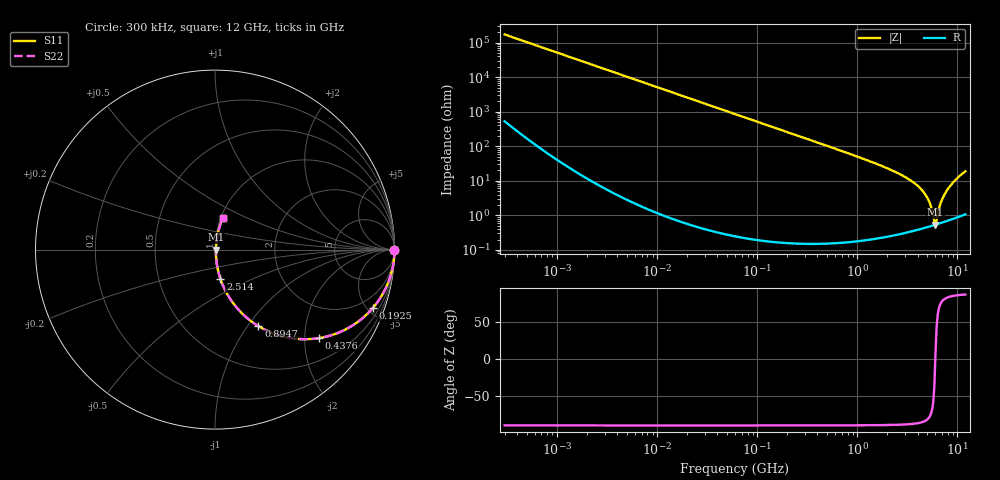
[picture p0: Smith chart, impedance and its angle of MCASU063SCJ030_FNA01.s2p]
! MCASU063SCJ030_FNA01  S-PARAMETER MODEL  ( Standard Model )
! Model Generated by TAIYO YUDEN Corporation (http://www.ty-top.com)
! Version 1.0
! TAIYO YUDEN Control No. 230609
! Copyright(c) 2023 TAIYO YUDEN CO.,LTD. All Rights Reserved.
! Product Description (link to TY-COMPAS)
! https://ds.yuden.co.jp/TYCOMPAS/or/detail?pn=MCASU063SCJ030BFNA01&u=M
! Products Name : Multilayer Ceramic Capacitors
! Characteristics :
!  Capacitance : 3 [pF] , Rated Voltage : 50 [V] , TCC : CJ / C0J
!  Case Size : 0.6 x 0.3 / 0.024 x 0.012 [mm/inch] , Thickness : 0.3 / 0.012 [mm/inch]
!  (Conditions: Temperature = 25 [degC] , DC Bias Voltage = 0 [V])
! External Node Assignments :
!  1  o---| |---o  2
! GND o---------o GND
! Frequency Range : 0.3MHz  -  12000MHz  [ 401 STEP ]
# MHZ S RI R 50
! Freq[MHz].  S11 Real  S11 Imag  S21 Real  S21 Imag  S12 Real  S12 Imag  S22 Real  S22 Imag
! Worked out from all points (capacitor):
!   401 points, 300 kHz to 12 GHz, reference 50 ohm
!   read as one part in series: C = 3.08 pF near 316.3 kHz
!   lowest |Z| = 538 mohm at 6.026 GHz (marker M1)
!   series resonance near 6.009 GHz, so ESL is about 230 pH
!   S11 on the Smith chart (normalised r, x): 300 kHz: open; 192.5 MHz: 1.00, -5.36; 437.6 MHz: 1.00, -2.35; 894.7 MHz: 1.00, -1.13; 2.514 GHz: 1.01, -0.34; 12 GHz: 1.02, +0.38
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0.3  1 -0.000581  2.12e-06 0.000581  2.12e-06 0.000581  1 -0.000581
1.769972  1 -0.00343  1.34e-05 0.00343  1.34e-05 0.00343  1 -0.00343
10.44266  0.9996 -0.0202  0.000413 0.0202  0.000413 0.0202  0.9996 -0.0202
60  0.9866 -0.1147  0.0134 0.1147  0.0134 0.1147  0.9866 -0.1147
192.4766  0.8776 -0.3274  0.1224 0.3274  0.1224 0.3274  0.8776 -0.3274
353.9943  0.6786 -0.4665  0.3214 0.4665  0.3214 0.4665  0.6786 -0.4665
437.5599  0.5794 -0.493  0.4206 0.493  0.4206 0.493  0.5794 -0.493
894.6982  0.2422 -0.4269  0.7578 0.4269  0.7578 0.4269  0.2422 -0.4269
2088.533  0.0473 -0.2066  0.9527 0.2066  0.9527 0.2066  0.0473 -0.2066
2514.07  0.0305 -0.1639  0.9695 0.1639  0.9695 0.1639  0.0305 -0.1639
3547.679  0.0123 -0.0934  0.9877 0.0934  0.9877 0.0934  0.0123 -0.0934
4502.883  0.00666 -0.0499  0.9933 0.0499  0.9933 0.0499  0.00666 -0.0499
5140.631  0.00536 -0.0268  0.9946 0.0268  0.9946 0.0268  0.00536 -0.0268
5420.343  0.00517 -0.0177  0.9948 0.0177  0.9948 0.0177  0.00517 -0.0177
5715.274  0.00516 -0.00868  0.9948 0.00868  0.9948 0.00868  0.00516 -0.00868
6026.253  0.00533 0.000513  0.9947 -0.000513  0.9947 -0.000513  0.00533 0.000513
6354.153  0.00568 0.00954  0.9943 -0.00954  0.9943 -0.00954  0.00568 0.00954
6699.894  0.00623 0.0191  0.9938 -0.0191  0.9938 -0.0191  0.00623 0.0191
7064.448  0.00702 0.0292  0.993 -0.0292  0.993 -0.0292  0.00702 0.0292
7854.144  0.0095 0.0515  0.9905 -0.0515  0.9905 -0.0515  0.0095 0.0515
9708.23  0.0203 0.1078  0.9797 -0.1078  0.9797 -0.1078  0.0203 0.1078
12000  0.0436 0.1776  0.9564 -0.1776  0.9564 -0.1776  0.0436 0.1776
